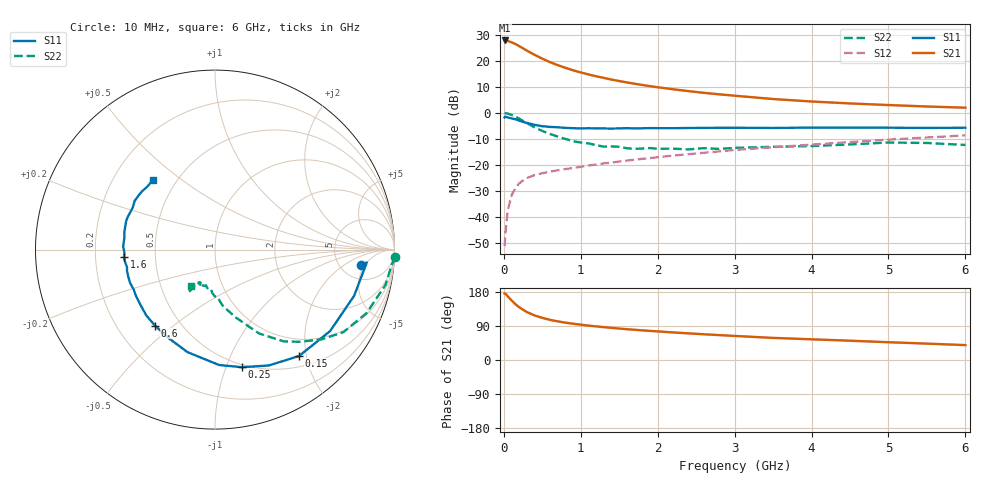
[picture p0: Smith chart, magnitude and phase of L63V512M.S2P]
!  INFINEON TECHNOLOGIES Small Signal Semiconductors
! BFR380L3 , Si-NPN RF-Transistor in TSLP-3-1
!  Vce=3.5 V,  Ic=12.5 mA
! Common Emitter S-Parameters:  07. March 2005
#  GHz  S  MA  R  50
! f  S11  S21  S12  S22
! GHz  Mag  Ang  Mag  Ang  Mag  Ang  Mag  Ang
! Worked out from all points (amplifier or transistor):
!   36 points, 10 MHz to 6 GHz, reference 50 ohm
!   highest |S21| = 27.8 dB at 10 MHz (marker M1)
!   |S21| within 3 dB of that: start of sweep to 249 MHz
!   unconditionally stable (mu >= 1): 2.222 GHz to 4.75 GHz
!   at 250 MHz: K = 0.27, MSG = 25.3 dB, |S12| = -25.9 dB
!   at 1.4 GHz: K = 0.89, MSG = 15.9 dB, |S12| = -19.1 dB
!   at 6 GHz: K = 0.96, MSG = 5.3 dB, |S12| = -8.6 dB
!   S11 on the Smith chart (normalised r, x): 10 MHz: 7.77, -4.05; 150 MHz: 0.68, -1.87; 250 MHz: 0.48, -1.14; 600 MHz: 0.36, -0.43; 1.6 GHz: 0.33, -0.04; 6 GHz: 0.37, +0.40
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0.01  0.8166 -6.1  24.41 175.7  0.0028 81.7  1.006 -2.4
0.02  0.8491 -4.8  24.37 175.3  0.0048 87.4  0.9884 -4.8
0.05  0.8167 -18.4  23.86 168.1  0.0133 82.6  0.9702 -11.7
0.1  0.7858 -35.3  22.5 157.3  0.0263 74.3  0.9159 -22.7
0.15  0.7555 -51.7  20.9 147.4  0.0363 66.7  0.8507 -32.7
0.2  0.7118 -65.1  19.01 139.1  0.0449 61.7  0.7763 -40.1
0.25  0.6725 -77.0  17.25 132.5  0.0507 57.0  0.6989 -47.3
0.3  0.6434 -88.0  15.58 126.5  0.0565 54.3  0.6398 -53.1
0.4  0.5913 -105.1  12.95 117.5  0.0644 50.5  0.528 -62.3
0.5  0.5564 -117.9  10.94 111.2  0.0699 48.8  0.4508 -67.6
0.6  0.5393 -128.3  9.373 105.9  0.0749 48.5  0.3954 -73.0
0.8  0.5169 -143.5  7.305 98.5  0.084 49.4  0.3173 -81.9
0.9  0.5099 -149.9  6.546 95.7  0.0879 50.1  0.2865 -84.9
1.1  0.5082 -158.4  5.453 90.7  0.0982 52.0  0.2606 -90.2
1.4  0.4999 -168.8  4.347 84.9  0.1115 54.3  0.228 -96.4
1.6  0.5094 -175.3  3.833 81.2  0.1222 55.5  0.2104 -103.5
2.2  0.5092 172.5  2.836 72.7  0.1521 58.4  0.2067 -108.9
2.8  0.5197 162.2  2.268 65.7  0.183 60.4  0.2043 -116.6
3.5  0.5148 152.8  1.844 58.3  0.2194 60.2  0.2246 -118.3
4.5  0.5222 145.8  1.518 50.9  0.2764 60.5  0.2488 -120.3
5.5  0.5151 137.0  1.326 43.2  0.3381 58.4  0.2653 -121.7
6  0.52 131.5  1.258 39.3  0.3708 56.8  0.2431 -123.0
